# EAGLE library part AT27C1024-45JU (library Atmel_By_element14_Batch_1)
EPROM
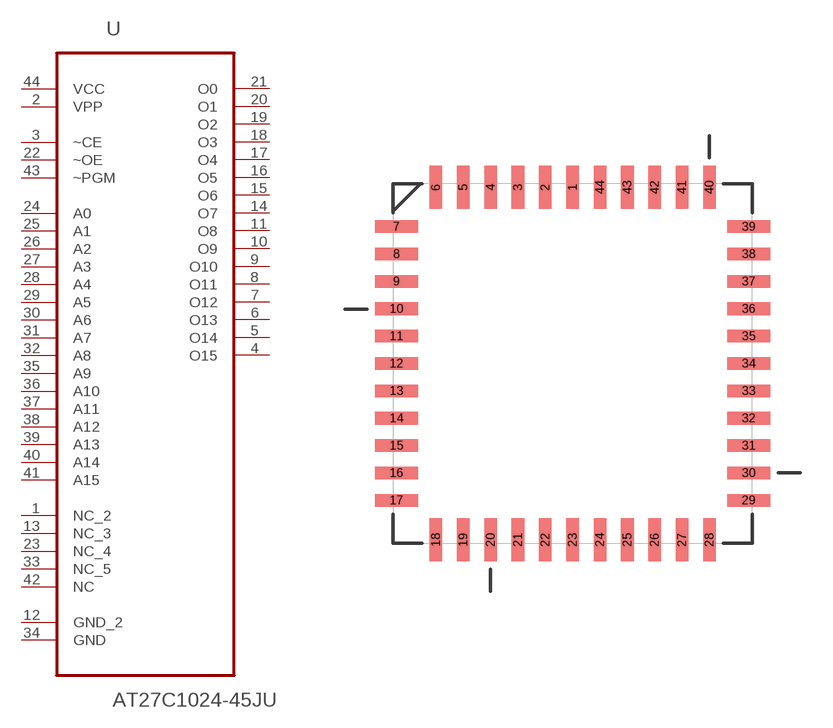
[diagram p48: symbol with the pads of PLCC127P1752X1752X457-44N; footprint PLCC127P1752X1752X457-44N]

Designator prefix U

## AT27C1024-45JU (DESCRIPTION: EPROM; MPN: AT27C1024-45JU; OC_FARNELL: 1841586; OC_NEWARK: 12T1362; PACKAGE: PLCC-44; SUPPLIER: Atmel)  [PLCC127P1752X1752X457-44N]
1  NC_2  nc
2  VPP  pwr
3  ~CE  in
4  O15  out
5  O14  out
6  O13  out
7  O12  out
8  O11  out
9  O10  out
10  O9  out
11  O8  out
12  GND_2  pas
13  NC_3  nc
14  O7  out
15  O6  out
16  O5  out
17  O4  out
18  O3  out
19  O2  out
20  O1  out
21  O0  out
22  ~OE  in
23  NC_4  nc
24  A0  in
25  A1  in
26  A2  in
27  A3  in
28  A4  in
29  A5  in
30  A6  in
31  A7  in
32  A8  in
33  NC_5  nc
34  GND  pas
35  A9  in
36  A10  in
37  A11  in
38  A12  in
39  A13  in
40  A14  in
41  A15  in
42  NC  nc
43  ~PGM  in
44  VCC  pwr

## Footprint PLCC127P1752X1752X457-44N (pad centres in mm)
smd 0.584 x 2.007: 1 0,8.179; 2 -1.27,8.179; 3 -2.54,8.179; 4 -3.81,8.179; 5 -5.08,8.179; 6 -6.35,8.179; 18 -6.35,-8.179; 19 -5.08,-8.179; 20 -3.81,-8.179; 21 -2.54,-8.179; 22 -1.27,-8.179; 23 0,-8.179; 24 1.27,-8.179; 25 2.54,-8.179; 26 3.81,-8.179; 27 5.08,-8.179; 28 6.35,-8.179; 40 6.35,8.179; 41 5.08,8.179; 42 3.81,8.179; 43 2.54,8.179; 44 1.27,8.179
smd 2.007 x 0.584: 7 -8.179,6.35; 8 -8.179,5.08; 9 -8.179,3.81; 10 -8.179,2.54; 11 -8.179,1.27; 12 -8.179,0; 13 -8.179,-1.27; 14 -8.179,-2.54; 15 -8.179,-3.81; 16 -8.179,-5.08; 17 -8.179,-6.35; 29 8.179,-6.35; 30 8.179,-5.08; 31 8.179,-3.81; 32 8.179,-2.54; 33 8.179,-1.27; 34 8.179,0; 35 8.179,1.27; 36 8.179,2.54; 37 8.179,3.81; 38 8.179,5.08; 39 8.179,6.35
